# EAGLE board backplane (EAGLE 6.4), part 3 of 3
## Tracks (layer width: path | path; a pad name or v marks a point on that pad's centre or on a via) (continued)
VCC_BACKPLANE  (via drill 0.6, 1.2) (continued)
  Bottom 0.254: v117.47,64.26 v117.47,61.72 | v103.38,357.76 v103.38,359.54 | v97.28,362.97 v97.28,360.43 | v153.42,365.89 v153.42,363.6 | v114.43,306.83 v112.14,306.83 | v109.09,307.59 v106.81,307.59 | v105.03,308.1 v103.89,309.25 | v120.02,308.36 v117.73,308.36 | v127.38,309.37 v125.09,309.37 | v122.81,292.23 v122.81,295.02 | v122.56,327.02 v122.56,324.74 | v116.08,328.04 v116.08,324.1 | v110.74,328.04 v110.74,324.1 | v116.08,338.96 116.08,335.03 | v110.74,338.96 v110.74,334.9 | v116.08,345.06 v116.08,341.88 | v110.74,345.19 v110.74,341.88 | v121.92,338.96 v121.92,334.9 | v129.74,343.23 v128.13,344.85 | v138.68,350.14 v138.68,347.85 | v115.95,296.55 v115.95,290.58 | v132.21,292.23 v132.21,295.02 | v115.95,261.24 v115.95,257.3 | v122.56,258.19 v122.56,260.48 | v115.95,251.08 v115.95,247.14 | v122.56,248.03 v122.56,250.32 | v115.95,241.17 v115.95,237.49 | v122.56,241.17 v122.56,237.49 | v132.72,248.28 v132.72,250.57 | v132.72,239.01 v132.72,240.79 | v132.72,258.19 v132.72,260.48 | v115.95,235.08 v115.95,231.39 | v122.56,235.08 v122.56,231.39 | v159.26,72.39 v157.23,74.42 | v101.53,144.53 v99.24,144.53 | v96.45,144.53 v94.16,144.53 | v101.53,115.83 v99.24,115.83 | v96.45,115.83 v94.16,115.83 | v165.35,163.19 v165.35,160.4
  Bottom 1.27: v235.08,187.58 v237.62,185.04 | v163.61,131.08 v163.61,124.69 | v134.35,118.65 v137.44,118.65 | v128,115.86 v131.09,115.86 | v123.43,120.69 v126.52,120.69 | v149.57,140.23 v143.98,140.23 | v162.18,243.21 v165.1,246.13 | v142.88,193.42 v142.88,196.72 143,196.85 | v183.51,87.5 v183.51,90.81 183.64,90.93 | v159.64,87.5 v159.64,90.81 159.77,90.93 | v146.27,35.08 v150.84,35.08 | v146.78,10.18 v150.84,10.18 | v165.32,46.25 v165.32,41.17 165.32,46.19 165.35,46.23 165.35,51.55 v165.32,51.59 | v163.29,55.65 v163.29,58.7 | v114.8,161.83 v114.8,156.75 | v88.63,156.75 v88.63,161.83 | v109.21,165.64 v111.49,167.93 | v36.6,90.71 39.14,90.71 v41.42,93 | v21.61,94.52 v21.61,99.1 | v13.74,94.52 v13.74,99.1 | v83.33,95.79 v83.33,93.13 | v60.73,93.13 v60.73,95.79 | v149.61,255.78 v152.65,258.83 | v69.36,291.37 v69.36,286.04 | v28.73,291.37 v28.73,285.53 | v92.48,198.16 v92.48,194.09 | v48.54,198.28 v48.54,193.97 | v165.1,253.49 v165.1,250.44 | v186.44,294.13 v186.44,289.05 | v151.38,294.13 v151.38,290.07 | v147.83,298.45 147.57,298.45 v145.29,300.74 | v137.92,280.67 v141.99,280.67 | v123.57,208.15 v127.89,208.15 | J4.13 42.39,181.84 v43.69,183.13 | v51.08,189.14 v48.28,186.34
  other vias: 116.08,334.9
  pour Top: 257.81,-3.81 -7.62,-3.81 -7.62,388.62 257.81,388.62
VCC_CONTROLLER  (via drill 1.2)
  Top 0.508: J4.2 57.73,168.73 59.18,170.18 59.18,178.05 63.5,182.37 63.5,191.52 65.02,193.04 TP22.TESTPOINT
  Top 1.27: v2.54,153.16 2.79,152.91 2.79,98.55 6.6,94.74 6.6,92.71 2.79,88.9 2.79,11.68 11.68,2.79 84.96,2.79 88.65,6.48 90.93,6.48 94.87,2.79 159.38,2.79 162.94,6.48 165.35,6.48 169.04,2.79 242.82,2.79 251.21,11.18 251.21,88.77 247.52,92.46 247.52,94.74 251.21,98.42 251.21,183.13 v246.76,187.58 | v246.63,193.04 234.95,204.72 234.95,249.88 J3.2
  Bottom 1.27: J4.2 57.63,168.63 57.66,165.1 45.72,153.16 v2.54,153.16 | v246.76,187.58 246.63,187.96 v246.63,193.04
VCC_LINUX  (via drill 0.6, 1.2)
  Top 0.508: v65.79,191.26 74.42,191.26 TP23.TESTPOINT
  Top 5.08: v8.38,184.15 v8.38,187.2 v8.38,190.25 v8.38,193.29 3.05,198.63 3.05,274.83 arc-47 6.35,282.45 arc48 8.89,287.4 arc48 6.35,292.61 arc-47 3.05,300.23 3.05,351.03 29.97,377.95 77.34,377.95 arc-47 84.96,374.65 arc39 89.92,372.11 arc42 95.12,374.65 arc-47 102.74,377.95 151.51,377.95 arc-47 159.13,374.65 arc39 164.08,372.11 arc42 169.29,374.65 arc-47 176.91,377.95 223.52,377.95 250.95,350.52 250.95,294.64 v237.49,281.18
  Bottom 0.508: J4.4 55.04,168.73 53.85,169.93 53.85,189.48 56.39,192.02 65.02,192.02 v65.79,191.26
  Bottom 1.27: J4.4 55.09,168.63 | J3.4 216.74,265.61 220.47,261.87
  Bottom 2.032: 55.09,168.63 51.82,164.85
  Bottom 5.08: 51.82,164.85 48.01,161.04 26.42,161.04 8.38,179.07 v8.38,184.15 v8.38,193.29 | 220.47,261.87 230.63,261.87 235.2,266.45 235.2,278.89 v237.49,281.18 v239.52,283.21 v241.55,285.24 v243.59,287.27
VSOL+
  Top 1.27: J8.1 37.08,151.64 32.77,155.96 32.77,169.27 J4.19
  Bottom 0.508: J4.19 34.72,171.27 34.04,171.96 34.04,186.18 TP12.TESTPOINT
VSOL-
  Top 1.27: J4.20 34.77,156.49 41.02,150.24 41.4,149.86 42.08,149.18 J8.2
  Bottom 0.508: J4.20 34.87,168.73 36.07,169.93 36.07,184.15 TP13.TESTPOINT

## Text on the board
tPlace: PPS | !BACK!- / !RESET | VCC / Back | GND | SDA | SCL | GND | VCC_MODn_METERED | VCC / Cont | VCC / Linux | VCC / Back | VSOL | VBATT | + | + | SMB / DATA | SMB / CLK | !SMB / !ALRT | GND | - | - | GND | + | VSOL | - | + | VBATT | - | Signpost Backplane | Pat Pannuto | Rev A. 2016-08-20
bPlace: + | VSOL | - | + | VBATT | -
